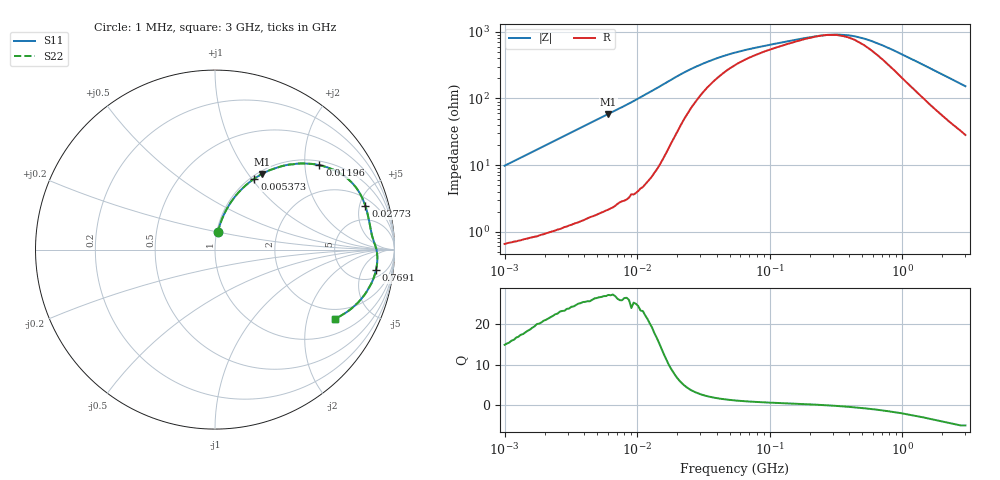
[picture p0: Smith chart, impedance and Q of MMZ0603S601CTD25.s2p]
! S-Parameter Data Generated by TDK Corporation
! Copyright(C) 2025 TDK Corporation.
! All Rights Reserved.
! TDK P/N: MMZ0603S601CTD25 (Chip Bead)
! Property: |Z|=600ohm at 100MHz
! Size(LxWxT): 0.6x0.3x0.3mm
! Model Type: s2p (Touchstone File Format Version 1.0)
! Frequency: DC=Yes Start=1MHz Stop=3000MHz 202points Log-sweep
! Model Generated on Feb. 6, 2025
! Terms and conditions regarding TDK Simulation Models:
! 1)This simulation model is being provided solely for informational
!  purposes. Please refer to the specifications of the products in
!  terms of detailed characteristics of such products.
! 2)In no event shall TDK Corporation of any of its subsidiaries be
!  liable for any loss or damage arising, directly or indirectly,
!  from any information contained in this simulation model, including,
!  but not limited to loss or damages arising from any inaccuracies,
!  omissions or errors in connection with such information.
! 3)Any and all copyrights on this simulation model are owned by
!  TDK Corporation.  Duplication or redistribution of this simulation
!  model without prior written permission from TDK Corporation
!  is prohibited.
! 4)This simulation model is subject to any modification or change
!  without any prior notice.
! 5)Neither TDK Corporation nor any of its subsidiaries shall make any
!  warranty, express or implied, including but not limited to the
!  correctness, implied warranties of merchantability and fitness for
!  a particular purpose with respect to this simulation models.
! 6)The use of this simulation model shall be deemed to have consented
!  to the terms and conditions hereof.
! Port Assignments:
!  1 ---@@@--- 2
! Applicable Conditions:
!  Temperature = 25 degC
!  DC Bias Current = 0 A
!  Small Signal Operation
# Hz S MA R 50
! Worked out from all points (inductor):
!   201 points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, 1 MHz to 3 GHz, reference 50 ohm
!   read as one part in series: L = 1.55 uH near 1.041 MHz
!   highest Q = 27.1 at 6.058 MHz (marker M1), where L = 1.53 uH
!   self-resonance near 263.3 MHz
!   S11 on the Smith chart (normalised r, x): 1 MHz: 1.01, +0.20; 5.373 MHz: 1.04, +1.03; 11.96 MHz: 1.11, +2.37; 27.73 MHz: 2.81, +5.71; 769.1 MHz: 8, -10; 3 GHz: 1.57, -3.00
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1000000  0.0967 80.6  0.9889 -5.5  0.9889 -5.5  0.0967 80.6
2226959  0.209 75.3  0.9683 -12.1  0.9683 -12.1  0.209 75.3
3900413  0.3474 67.4  0.9242 -20.3  0.9242 -20.3  0.3474 67.4
5372736  0.4523 61.0  0.8751 -26.9  0.8751 -26.9  0.4523 61.0
6058321  0.4958 58.2  0.8504 -29.7  0.8504 -29.7  0.4958 58.2
8686058  0.6322 48.6  0.7508 -39.2  0.7508 -39.2  0.6322 48.6
1.196486e7  0.748 39.0  0.6296 -48.3  0.6296 -48.3  0.748 39.0
1.461624e7  0.8073 32.6  0.5402 -53.7  0.5402 -53.7  0.8073 32.6
1.934349e7  0.8569 24.2  0.4137 -58.1  0.4137 -58.1  0.8569 24.2
2.773354e7  0.8726 16.1  0.2914 -56.3  0.2914 -56.3  0.8726 16.1
3.976269e7  0.8736 10.9  0.2181 -49.3  0.2181 -49.3  0.8736 10.9
5.477226e7  0.8744 7.8  0.1791 -41.7  0.1791 -41.7  0.8744 7.8
9.216659e7  0.8797 4.6  0.142 -29.8  0.142 -29.8  0.8797 4.6
2.136344e8  0.8955 1.0  0.1057 -8.3  0.1057 -8.3  0.8955 1.0
3.188066e8  0.9027 -1.0  0.09872 9.1  0.09872 9.1  0.9027 -1.0
4.219165e8  0.9057 -2.6  0.1038 23.4  0.1038 23.4  0.9057 -2.6
5.81181e8  0.9065 -4.8  0.1234 38.4  0.1234 38.4  0.9065 -4.8
7.691493e8  0.9041 -7.3  0.1542 48.0  0.1542 48.0  0.9041 -7.3
8.005644e8  0.9035 -7.7  0.1599 49.1  0.1599 49.1  0.9035 -7.7
1.645649e9  0.8678 -17.3  0.3093 56.4  0.3093 56.4  0.8678 -17.3
2.266846e9  0.828 -23.4  0.407 53.9  0.407 53.9  0.828 -23.4
3e9  0.7734 -29.8  0.5064 49.5  0.5064 49.5  0.7734 -29.8
